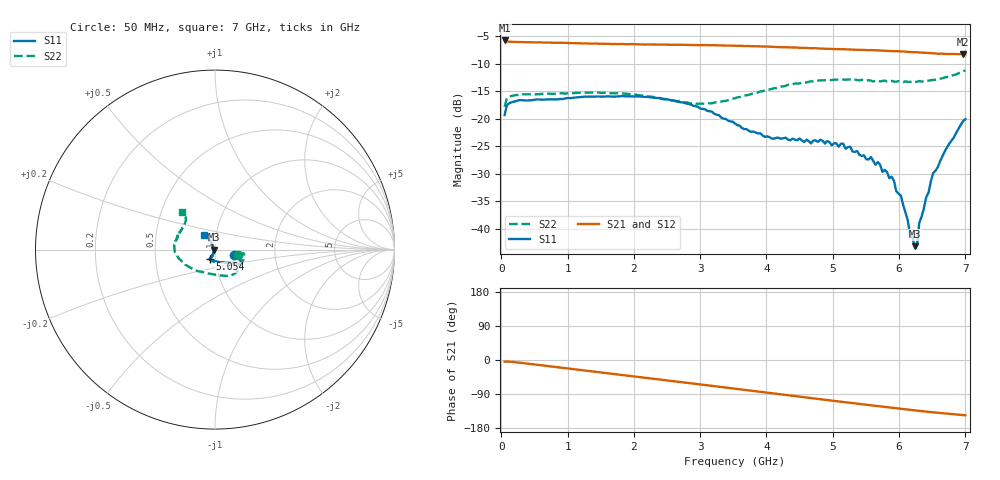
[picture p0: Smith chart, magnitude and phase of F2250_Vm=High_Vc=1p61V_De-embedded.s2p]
! Integrated Device Technology
! Corporate Headquarters
! 6024 Silver Creek Valley Road
! San Jose, CA 95138  USA
! Phone:  1-408-284-8200
! Toll Free:  1-800-223-1366
! Webpage:  http://www.idt.com/
! Timing and RF Division
! 515 Groton Road, Suite 102
! Westford, MA 01886-6024
! Device:  F2250
! Description: Voltage Variable RF Attenuator
! Frequency:  50.0 -  6000.00 MHz
! Package:  3x3 mm Thin QFN Plastic Package: 16 pin
! Ports:  2 RF, 3 DC
!  Pin  1  = GND
!  Pin  2  = NC
!  Pin  3  = RF1  = Port 1
!  Pin  4  = NC
!  Pin  5  = GND
!  Pin  6  = GND
!  Pin  7  = GND
!  Pin  8  = GND
!  Pin  9  = NC
!  Pin 10  = RF2  = Port 2
!  Pin 11  = NC
!  Pin 12  = GND
!  Pin 13  = GND
!  Pin 14  = VCNTRL
!  Pin 15  = VDD
!  Pin 16  = VMODE
! Vcntrl:  1.610 Volts
! Vmode:  +3.300 Volts
! Vdd:  +3.30  Volts
! Current:  1.329 mA
! Data:  The device was measured on a the F2250 evaluation board which has
!  individual transmission lines to the RF pins.  Data was collected
!  using a calibrated network analyzer.  The evaluation board was
!  de-embedded using a TRL calibration technique.
!  The reference plane is the edge of the package pin.
! Misc:  SN 10
!  Action Tracker AT0258
! Date Measured:  2014-11-26
! Date:  2015-10-15  MJV
! Note:
!  Integrated Device Technology supplies this data as a sample of measured
!  data at the package pin for this product.  Your particular data for this
!  product may vary.
!  Data was taken at 25 degrees C.
!  Integrated Device Technology reserves the right to change this data at anytime.
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# GHz S dB R 50
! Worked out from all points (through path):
!   201 points, 50 MHz to 7 GHz, reference 50 ohm
!   highest |S21| = -5.73 dB at 50 MHz (marker M1); lowest = -8.3 dB at 6.965 GHz (marker M2)
!   group delay of S21, straight-line fit = 58.5 ps
!   lowest |S11| = -43.2 dB at 6.236 GHz (marker M3), VSWR 1.01, Z = 49.3 - j0.124 ohm
!   |S11| at or under -10 dB: start of sweep to end of sweep
!   |S22| runs from -17.8 to -11.2 dB; largest |S21 - S12| = 0.0028
!   S11 on the Smith chart (normalised r, x): 50 MHz: 1.23, -0.07; 5.054 GHz: 0.94, -0.10; 7 GHz: 0.88, +0.14
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0.05  -19.30 -15.7  -5.73 -4.5  -5.73 -4.5  -17.80 -13.2
0.08475  -17.50 -8.3  -5.89 -4.0  -5.90 -4.0  -16.20 -8.1
0.2585  -16.64 -8.1  -6.01 -6.8  -6.04 -6.7  -15.63 -11.7
1.2315  -15.99 -25.7  -6.27 -27.3  -6.25 -27.3  -15.20 -42.8
2.37825  -16.22 -31.3  -6.46 -51.1  -6.46 -51.1  -16.14 -70.8
2.969  -17.84 -35.6  -6.57 -63.7  -6.58 -63.7  -17.27 -97.1
3.525  -20.85 -52.8  -6.68 -75.9  -6.69 -75.9  -16.24 -129.9
4.081  -23.59 -84.9  -6.89 -88.0  -6.90 -88.0  -14.54 -155.4
4.7065  -23.95 -114.3  -7.13 -101.3  -7.13 -101.4  -13.18 -174.0
5.054  -24.46 -116.2  -7.30 -108.7  -7.30 -108.7  -12.85 177.6
5.57525  -26.94 -116.6  -7.48 -119.4  -7.49 -119.5  -13.03 165.4
5.85325  -30.80 -113.0  -7.65 -125.1  -7.67 -125.2  -13.19 156.7
5.888  -30.52 -116.2  -7.67 -125.9  -7.68 -126.0  -13.08 156.8
5.9575  -33.16 -110.9  -7.67 -127.3  -7.68 -127.4  -13.24 154.0
6.027  -33.97 -118.7  -7.73 -128.7  -7.74 -128.8  -13.27 152.6
6.166  -41.12 -130.6  -7.83 -131.5  -7.82 -131.6  -13.27 147.4
6.2355  -43.17 -169.6  -7.87 -132.8  -7.86 -133.0  -13.27 145.8
6.27025  -42.94 162.9  -7.87 -133.6  -7.89 -133.6  -13.25 144.1
6.305  -38.91 138.0  -7.92 -134.3  -7.94 -134.3  -13.11 143.1
6.5135  -29.84 118.8  -8.06 -138.0  -8.07 -138.2  -12.91 136.8
6.96525  -20.44 127.0  -8.25 -145.4  -8.28 -145.5  -11.34 131.9
7  -20.05 127.4  -8.25 -145.9  -8.27 -146.0  -11.17 131.1
